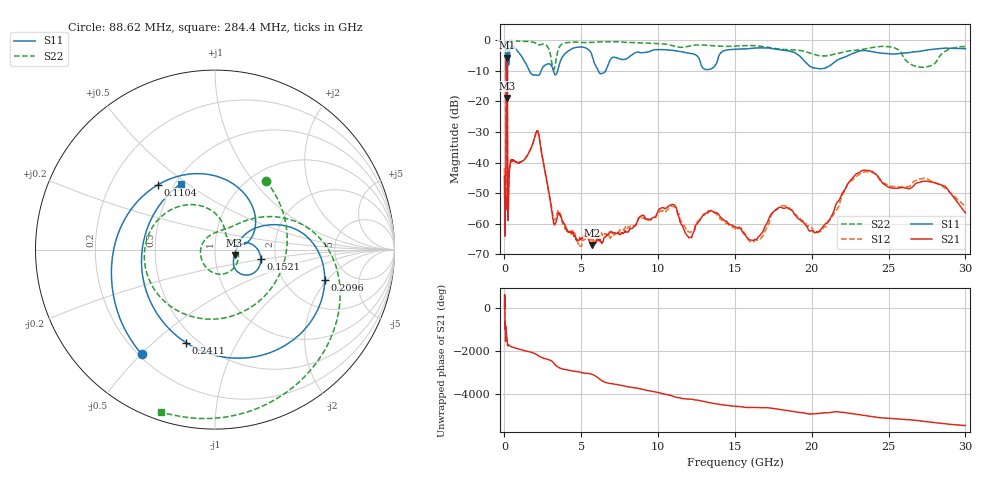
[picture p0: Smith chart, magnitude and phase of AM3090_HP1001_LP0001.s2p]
! Date/Time: Thu, Feb 28, 2019 2:02 PM
! Network Analyzer: Agilent Technologies E8364B Rev: A.07.50.67
! Sweep from 0.010 to 30.000 GHz, 1601 Points, Sweep Type: LOG
! Power Supply: 5.023 V, 0.002 A
# Hz S DB R 50
!freq MagS11 AngS11 MagS21 AngS21 MagS12 AngS12 MagS22 AngS22
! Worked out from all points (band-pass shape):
!   1601 points, 10 MHz to 30 GHz, reference 50 ohm
!   highest |S21| = -5.72 dB at 144.7 MHz (marker M1); lowest = -66.9 dB at 5.697 GHz (marker M2)
!   |S21| within 3 dB of the highest: 122.8 MHz to 180.7 MHz (57.92 MHz wide, 38.2 % of centre)
!   lowest |S11| = -18.9 dB at 180.3 MHz (marker M3), VSWR 1.25, Z = 62.1 - j3.86 ohm
!   |S11| at or under -10 dB: 1.609 GHz to 2.387 GHz (777.8 MHz wide, 38.9 % of centre); 3.186 GHz to 3.462 GHz (275.9 MHz wide, 8.3 % of centre); 6.102 GHz to 6.589 GHz (488 MHz wide, 7.69 % of centre)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
!   |S22| runs from -22.2 to -0.1 dB; largest |S21 - S12| = 0.012
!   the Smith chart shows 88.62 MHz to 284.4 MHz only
!   S11 on the Smith chart (normalised r, x): 88.62 MHz: 0.21, -0.50; 110.4 MHz: 0.41, +0.39; 152.1 MHz: 1.67, -0.18; 209.6 MHz: 3.31, -1.90; 241.1 MHz: 0.44, -0.64; 284.4 MHz: 0.53, +0.47
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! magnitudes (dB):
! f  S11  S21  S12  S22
! 10 MHz  -0.3  -48.6  -42.0  -0.5
! 38.04 MHz  -0.5  -59.7  -60.6  -1.3
! 48.37 MHz  -0.7  -51.2  -48.8  -1.5
! 88.62 MHz  -2.9  -50.3  -52.1  -6.4
! 110.4 MHz  -6.4  -20.1  -20.2  -7.9
! 144.7 MHz  -13.0  -5.7  -5.7  -17.9
! 152.1 MHz  -11.7  -5.8  -5.7  -16.7
! 180.3 MHz  -18.9  -8.6  -8.6  -19.2
! 192.5 MHz  -12.5  -17.5  -17.4  -10.4
! 209.6 MHz  -3.9  -49.3  -47.5  -2.5
! 241.1 MHz  -5.3  -55.0  -57.1  -0.7
! 284.4 MHz  -7.7  -47.5  -47.4  -0.4
! 550.5 MHz  -2.1  -39.3  -39.2  -0.2
! 2.084 GHz  -11.4  -29.9  -29.9  -1.2
! 3.236 GHz  -10.8  -60.3  -58.5  -9.4
! 5.697 GHz  -4.9  -66.9  -64.8  -0.8
! 7.926 GHz  -6.2  -62.7  -60.7  -0.8
! 10.7 GHz  -3.3  -54.2  -54.9  -1.5
! 11.95 GHz  -4.2  -64.1  -62.4  -2.1
! 20.31 GHz  -9.2  -62.8  -62.5  -4.9
! 23.48 GHz  -3.5  -42.5  -43.0  -2.9
! 30 GHz  -2.8  -56.4  -54.2  -2.1
